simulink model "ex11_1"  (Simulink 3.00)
settings: Solver=ode4  SolverMode=SingleTasking  StartTime=0.0  StopTime=50  FixedStep=0.0005  MaxStep=.0001  RelTol=1e-3  AbsTol=1e-6

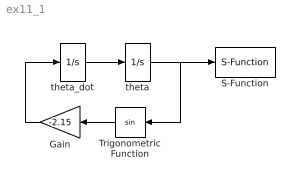
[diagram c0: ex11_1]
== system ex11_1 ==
  Gain : Gain  Orientation=left  Gain=-2.15  SaturateOnIntegerOverflow=on
  S-Function : S-Function  FunctionName=s_anm81s  PortCounts=[]  SFunctionModules=''
  Trigonometric Function : Trigonometry  Orientation=left  Operator=sin  OutputSignalType=auto
  theta : Integrator  ExternalReset=none  InitialConditionSource=internal  InitialCondition=1  LimitOutput=off  UpperSaturationLimit=inf  LowerSaturationLimit=-inf  ShowSaturationPort=off  ShowStatePort=off  AbsoluteTolerance=auto
  theta_dot : Integrator  ExternalReset=none  InitialConditionSource=internal  InitialCondition=0  LimitOutput=off  UpperSaturationLimit=inf  LowerSaturationLimit=-inf  ShowSaturationPort=off  ShowStatePort=off  AbsoluteTolerance=auto
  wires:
  theta/1 -> S-Function/1, Trigonometric Function/1
  Gain/1 -> theta_dot/1
  Trigonometric Function/1 -> Gain/1
  theta_dot/1 -> theta/1
